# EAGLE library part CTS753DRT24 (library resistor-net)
Network Resistor CTS 753 Series Leadless Surface Mount Source: http://www.ctscorp.com/components/Datasheets/753.pdf Distributor: Digi Key
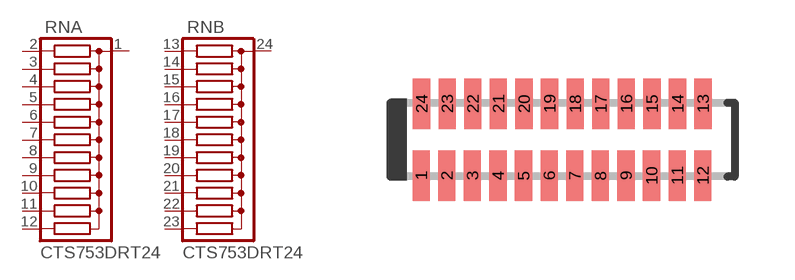
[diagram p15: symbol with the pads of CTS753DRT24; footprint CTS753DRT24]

Designator prefix RN; gates A=RN1X11 B=RN1X11

## CTS753DRT24 (OC_FARNELL: unknown; OC_NEWARK: unknown)  [CTS753DRT24]
1  A:C  pas
2  A:1  pas
3  A:2  pas
4  A:3  pas
5  A:4  pas
6  A:5  pas
7  A:6  pas
8  A:7  pas
9  A:8  pas
10  A:9  pas
11  A:10  pas
12  A:11  pas
13  B:1  pas
14  B:2  pas
15  B:3  pas
16  B:4  pas
17  B:5  pas
18  B:6  pas
19  B:7  pas
20  B:8  pas
21  B:9  pas
22  B:10  pas
23  B:11  pas
24  B:C  pas

## Footprint CTS753DRT24 (pad centres in mm)
Network Resistor Leadless Surface Mount Series 753 Source: http://www.ctscorp.com/components/Datasheets/753.pdf
smd 0.43 x 1.27: 1 -3.525,-0.9; 2 -2.885,-0.9; 3 -2.245,-0.9; 4 -1.605,-0.9; 5 -0.965,-0.9; 6 -0.325,-0.9; 7 0.315,-0.9; 8 0.955,-0.9; 9 1.595,-0.9; 10 2.235,-0.9; 11 2.875,-0.9; 12 3.515,-0.9; 13 3.52,0.9; 14 2.885,0.9; 15 2.245,0.9; 16 1.605,0.9; 17 0.965,0.9; 18 0.325,0.9; 19 -0.315,0.9; 20 -0.955,0.9; 21 -1.595,0.9; 22 -2.235,0.9; 23 -2.875,0.9; 24 -3.515,0.9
